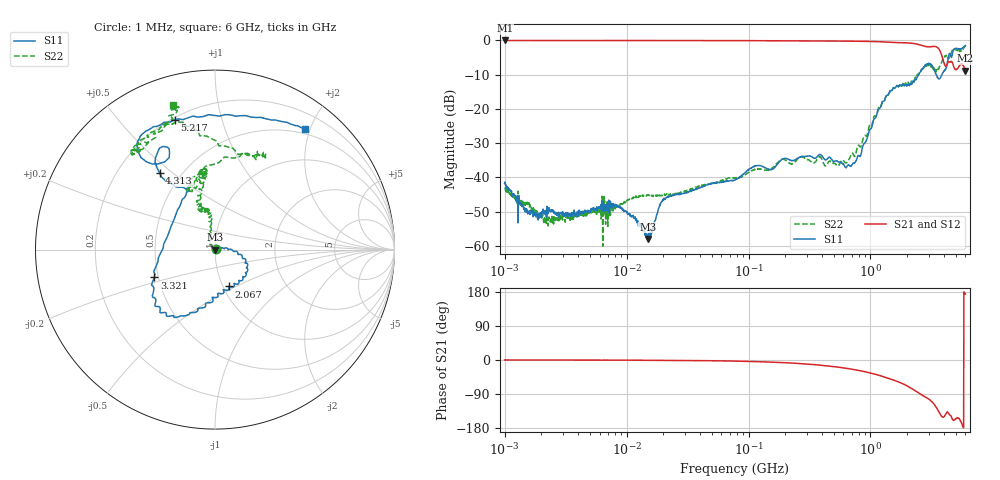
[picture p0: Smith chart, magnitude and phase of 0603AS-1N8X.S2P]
!s-Parameter Generated by FASTRON Sdn. Bhd.
!FASTRON P/N : 0603AS-1N8X
!Keysight Technologies: E5071C_MY46733604_B.14.02
!Date: Tue Nov 21 14:53:13 2023
!Version  :Rev01  Tue Nov 21 14:53:13 2023
!Data & Calibration Information:
!Freq  S11:SOLT2(ON)  S21:SOLT2(ON)  S12:SOLT2(ON)  S22:SOLT2(ON)
!PortZ  Port1:50+j0  Port2:50+j0
!When reading reference impedance value at option line is always used.
! Remarks : This data is being provided solely for informational purposes.
# Hz S dB R 50
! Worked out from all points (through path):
!   1601 points, 1 MHz to 6 GHz, reference 50 ohm
!   highest |S21| = -0.02 dB at 1.006 MHz (marker M1); lowest = -8.8 dB at 6 GHz (marker M2)
!   group delay of S21, straight-line fit = 91.4 ps
!   lowest |S11| = -58.0 dB at 14.93 MHz (marker M3), VSWR 1.00, Z = 50.1 - j0.0101 ohm
!   |S11| at or under -10 dB: start of sweep to 2.481 GHz; 3.473 GHz to 3.854 GHz (380.7 MHz wide, 10.4 % of centre)
!   |S22| runs from -60.1 to -1.5 dB; largest |S21 - S12| = 0.0076
!   S11 on the Smith chart (normalised r, x): 1 MHz: 1.02, +0.01; 2.067 GHz: 1.07, -0.46; 3.321 GHz: 0.48, -0.17; 4.313 GHz: 0.38, +0.45; 5.217 GHz: 0.21, +0.72; 6 GHz: 0.43, +1.93
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1000000  -41.76 19.7  -0.03 0.1  -0.05 0.2  -43.22 25.0
1006392  -41.36 17.6  -0.02 0.1  -0.04 0.2  -43.19 21.4
1819981  -50.44 9.8  -0.04 -0.0  -0.04 0.0  -49.44 -1.5
4277066  -50.56 27.1  -0.04 -0.2  -0.04 -0.1  -51.08 35.8
8345722  -48.23 32.5  -0.04 -0.4  -0.04 -0.3  -48.65 33.8
1.493236e7  -57.97 -4.6  -0.04 -0.6  -0.05 -0.6  -45.11 21.1
1.823719e7  -49.21 29.3  -0.04 -0.8  -0.05 -0.7  -45.22 35.8
2.231736e7  -45.62 35.1  -0.05 -0.9  -0.05 -0.8  -44.97 46.4
7.757876e7  -40.72 44.4  -0.06 -2.9  -0.07 -2.9  -40.11 42.6
1.886184e8  -34.72 57.5  -0.10 -6.8  -0.11 -6.8  -34.73 64.3
3.307917e8  -33.93 44.7  -0.14 -11.6  -0.15 -11.6  -35.55 77.2
7.165695e8  -35.92 23.9  -0.23 -24.7  -0.24 -24.7  -33.02 145.5
1.414819e9  -15.47 -17.2  -0.52 -48.7  -0.52 -48.7  -15.61 96.6
2.066863e9  -13.14 -68.8  -0.76 -70.9  -0.77 -71.0  -12.73 111.8
2.819297e9  -7.12 -120.9  -1.79 -97.7  -1.78 -97.7  -7.14 98.4
3.320724e9  -8.60 -155.3  -1.73 -116.3  -1.71 -116.5  -8.55 109.1
3.705459e9  -11.08 147.8  -2.96 -141.2  -2.95 -141.6  -7.51 106.9
4.090194e9  -8.52 115.2  -7.35 -145.6  -7.37 -145.9  -4.60 66.5
4.312935e9  -5.58 125.9  -6.42 -138.5  -6.44 -138.8  -5.18 65.5
4.880806e9  -2.43 123.5  -8.12 -158.1  -8.16 -158.3  -2.63 114.8
5.216564e9  -2.40 107.2  -8.09 -153.3  -8.13 -153.3  -2.89 128.1
6e9  -1.53 53.0  -8.82 174.3  -8.80 174.4  -1.54 106.3
